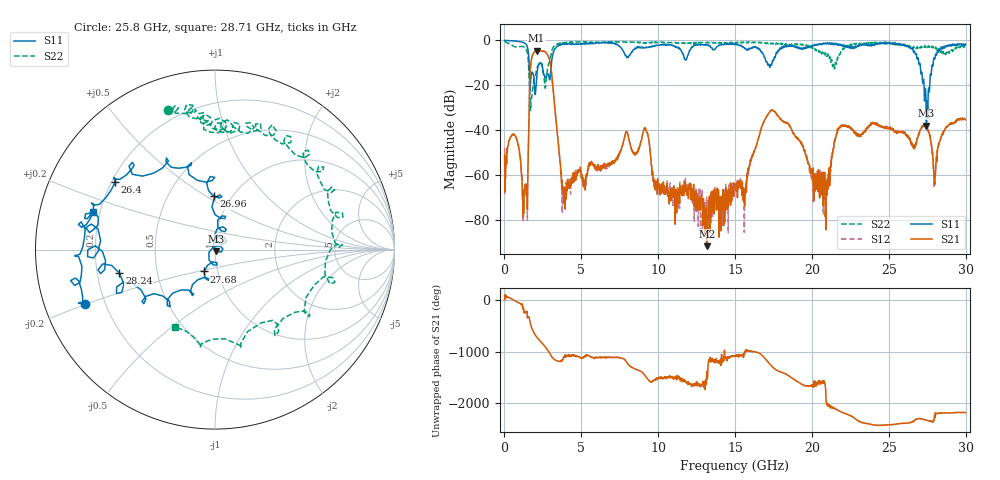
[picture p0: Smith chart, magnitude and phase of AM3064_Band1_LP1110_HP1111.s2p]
# Hz S DB R 50.0
!freq dBS11 angS11 dBS21 angS21 dBS12 angS12 dBS22 angS22
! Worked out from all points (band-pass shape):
!   1600 points, 10 MHz to 29.98 GHz, reference 50 ohm
!   highest |S21| = -4.54 dB at 2.091 GHz (marker M1); lowest = -91.9 dB at 13.19 GHz (marker M2)
!   |S21| within 3 dB of the highest: 1.784 GHz to 2.885 GHz (1.101 GHz wide, 47.2 % of centre)
!   lowest |S11| = -38.1 dB at 27.45 GHz (marker M3), VSWR 1.03, Z = 50.8 - j0.997 ohm
!   |S11| at or under -10 dB: 1.6 GHz to 2.307 GHz (707.6 MHz wide, 36.2 % of centre); 2.324 GHz to 3.056 GHz (731.7 MHz wide, 27.2 % of centre); 26.95 GHz to 27.89 GHz (939.2 MHz wide, 3.42 % of centre)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
!   |S22| runs from -31.3 to -0.4 dB; largest |S21 - S12| = 0.011
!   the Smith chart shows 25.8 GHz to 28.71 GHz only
!   S11 on the Smith chart (normalised r, x): 25.8 GHz: 0.13, -0.20; 26.4 GHz: 0.21, +0.29; 26.96 GHz: 0.83, +0.54; 27.68 GHz: 0.86, -0.21; 28.24 GHz: 0.30, -0.11; 28.71 GHz: 0.17, +0.15
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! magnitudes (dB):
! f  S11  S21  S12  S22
! 10 MHz  0.0  -50.9  -47.9  -0.4
! 1.341 GHz  -1.4  -64.9  -64.4  -3.1
! 1.753 GHz  -15.1  -8.5  -8.5  -25.9
! 2.091 GHz  -17.3  -4.5  -4.6  -13.0
! 2.953 GHz  -17.4  -9.2  -9.2  -9.1
! 3.834 GHz  -1.6  -68.3  -70.9  -1.1
! 5.015 GHz  -1.6  -61.1  -59.6  -0.7
! 9.157 GHz  -3.4  -39.2  -39.1  -1.1
! 10 GHz  -2.2  -65.8  -65.8  -0.9
! 13.19 GHz  -1.8  -91.9  -71.6  -1.1
! 15 GHz  -1.9  -64.6  -66.0  -1.3
! 17.39 GHz  -10.7  -31.2  -31.2  -1.5
! 19.99 GHz  -2.7  -59.1  -60.9  -3.1
! 25 GHz  -1.1  -39.5  -39.2  -1.1
! 25.8 GHz  -2.1  -40.7  -40.8  -1.7
! 26.4 GHz  -3.5  -44.5  -45.5  -2.9
! 26.96 GHz  -10.5  -41.2  -41.2  -3.0
! 27.45 GHz  -38.1  -38.6  -38.8  -2.4
! 27.68 GHz  -17.3  -42.3  -42.9  -2.6
! 28.24 GHz  -5.2  -46.0  -47.0  -4.8
! 28.71 GHz  -2.9  -39.1  -38.6  -6.3
! 29.98 GHz  -1.6  -35.5  -34.9  -2.8
